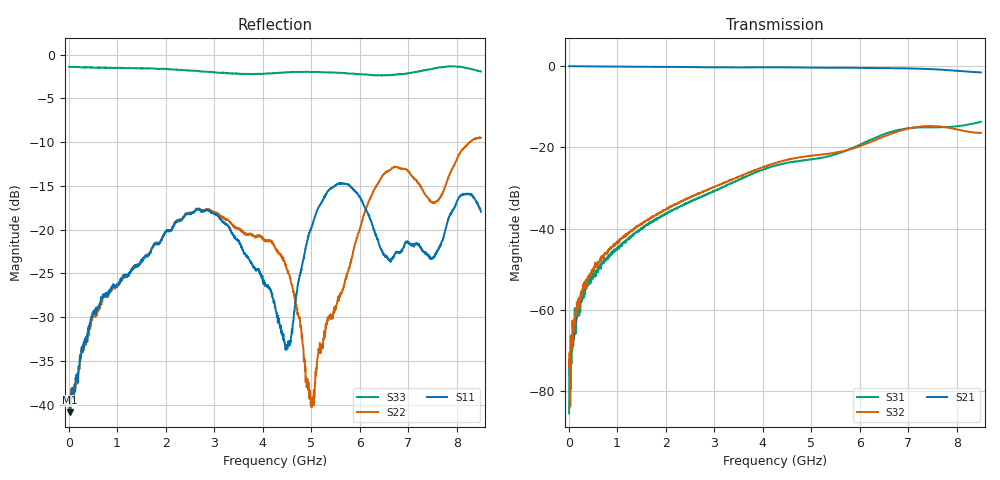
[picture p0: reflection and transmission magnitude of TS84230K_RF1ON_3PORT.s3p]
! Created with skrf (http://scikit-rf.org).
# Hz S RI R 50.0
!freq ReS11 ImS11 ReS12 ImS12 ReS13 ImS13
! ReS21 ImS21 ReS22 ImS22 ReS23 ImS23
! ReS31 ImS31 ReS32 ImS32 ReS33 ImS33
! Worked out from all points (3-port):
!   1601 points, 10 MHz to 8.5 GHz, reference 50 ohm
!   strongest paths, dB at 10 MHz, 2.132 GHz, 4.255 GHz, 6.378 GHz, 8.5 GHz:
!     S21: -0.1, -0.3, -0.4, -0.6, -1.6
!     S32: -72.3, -34.4, -23.9, -17.9, -16.5
!     S31: -85.4, -35.6, -24.6, -17.4, -13.7
!   lowest |S11| = -40.9 dB at 25.92 MHz (marker M1), VSWR 1.02, Z = 50.9 - j0.0675 ohm
!   |S11| at or under -10 dB: start of sweep to end of sweep
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1e7  0.0104 -0.00262  0.9885 -0.0054  0.000408 4.16e-06
     0.988 -0.00498  0.0102 -0.00259  0.000145 5.69e-05
     -3.65e-05 3.97e-05  -0.000239 4.79e-05  -0.8507 0.00516
2.591875e7  0.00903 -0.000663  0.9888 -0.00916  1.95e-05 7.29e-05
            0.9884 -0.00892  0.00943 -0.000879  0.00021 3.65e-05
            0.000114 8.51e-05  0.000122 0.000157  -0.8491 0.0087
2.169438e8  0.00967 -0.0134  0.9836 -0.078  0.000112 0.00106
            0.9833 -0.0778  0.0096 -0.0131  0.000297 0.00142
            0.000205 0.000824  8.99e-05 0.00116  -0.8462 0.0741
7.369562e8  -0.00152 -0.0425  0.9466 -0.2542  -0.000679 0.00383
            0.9461 -0.2535  -0.00487 -0.0421  -6.54e-05 0.00491
            -0.000573 0.00402  -0.00014 0.00486  -0.8066 0.2443
2.673738e9  -0.1059 -0.0772  0.5693 -0.7748  -0.00123 0.0236
            0.5696 -0.7739  -0.0948 -0.0909  0.0081 0.0257
            -0.00123 0.0238  0.00817 0.0256  -0.3753 0.7116
4.255e9  -0.0228 -0.0281  0.0684 -0.9562  0.0231 0.0544
         0.0695 -0.9556  -0.0161 -0.0767  0.0497 0.0397
         0.023 0.0545  0.0495 0.0399  0.3542 0.6983
4.536231e9  -0.0211 0.0081  -0.0351 -0.9565  0.0326 0.0558
            -0.0327 -0.9567  -0.0204 -0.052  0.0614 0.0354
            0.0324 0.0559  0.0612 0.0356  0.4924 0.62
5.029712e9  0.0155 0.1069  -0.2112 -0.9259  0.0452 0.0553
            -0.2105 -0.926  -0.00597 0.00789  0.0763 0.0214
            0.0452 0.0555  0.076 0.0213  0.654 0.4521
6.4624e9  0.0674 -0.0349  -0.6728 -0.6523  0.1227 0.0701
          -0.6715 -0.6527  -0.0513 -0.1951  0.1301 -0.027
          0.1225 0.07  0.1299 -0.0264  0.7583 -0.0569
8.5e9  -0.00365 -0.1265  -0.8117 0.1794  0.1807 -0.0996
       -0.8108 0.1757  0.1734 -0.2854  -0.0039 -0.1504
       0.1804 -0.0987  -0.00336 -0.15  0.2279 -0.7664
